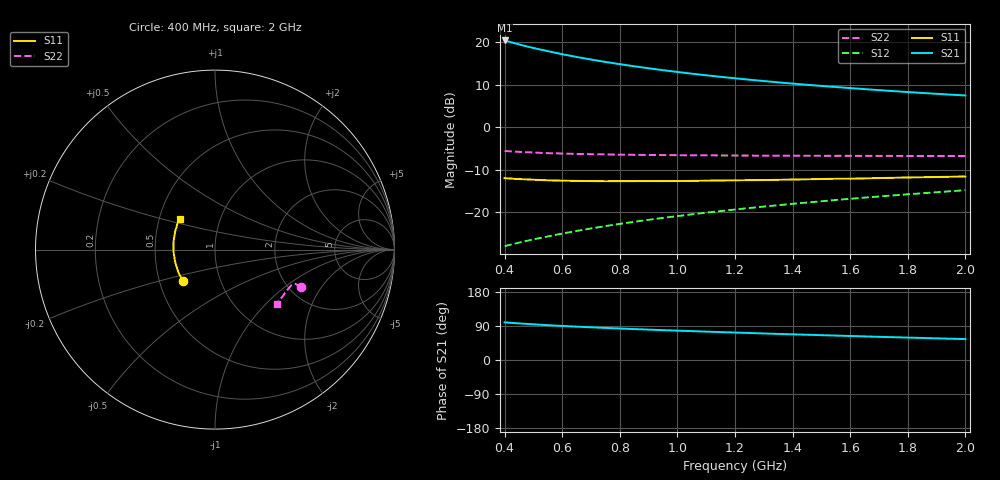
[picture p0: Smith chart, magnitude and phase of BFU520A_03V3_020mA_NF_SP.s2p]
! Filename:  P:\Prog\Test\Noise\ATS_data\Testdata_Net\06 Compressed Noise after Statistics\BFU520A_APG2013_30_A05_03p3V_020mA_NF_CM01_D.sf
! Date/Time: Wed 24/Apr/2013 20:06:17
! BFU520A_APG2013_30_A05_03p3V_1to20mA_NF_CM01_Bias8_R.sf
! Noise Parameter Data File
! BFU520A_APG2013_30_A05_03p3V_1to20mA_NF_CM01
! Date/time: Thu Apr 11 00:04:13 2013
! VAR V_out= 3.301000
! VAR I_out= 19.995000
! VAR V_in= 0.862000
! VAR I_in= 0.236350
! Device data file deembeded for feedlines and parallel
! Original file: \06 Compressed Noise after Statistics\BFU520A_APG2013_30_A05_03p3V_020mA_NF_CM01_R.sf
! Feed-files: PR017V01_150413_Feed1.s2p, PR017V01_150413_Feed2.s2p
! Parallel-file: PR017V01_150413_Par.s2p
# MHz S MA R 50
!  Freq-MHz  S11-mag  S11-arg  S21-mag  S21-arg  S12-mag  S12-arg  S22-mag  S22-arg
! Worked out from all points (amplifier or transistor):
!   37 points, 400 MHz to 2 GHz, reference 50 ohm
!   highest |S21| = 20.4 dB at 400 MHz (marker M1)
!   |S21| within 3 dB of that: start of sweep to 583.6 MHz
!   unconditionally stable (mu >= 1): 665.9 MHz to 1.644 GHz
!   at 500 MHz: K = 0.96, MSG = 22.5 dB, |S12| = -26.5 dB
!   at 1.1 GHz: K = 1.02, MAG = 15.3 dB, |S12| = -20.2 dB
!   at 2 GHz: K = 0.98, MSG = 11.2 dB, |S12| = -14.9 dB
!   lowest NFmin = 1.13 dB at 420 MHz
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400  0.2501 -136.2  10.45 99.4  0.03959 72.2  0.5229 -23.6
420  0.2478 -138.8  10 98.2  0.04118 72.5  0.5172 -23.5
440  0.245 -141.4  9.591 97.1  0.04278 72.8  0.5126 -23.4
460  0.2431 -143.7  9.207 96.1  0.04435 73.1  0.5084 -23.3
480  0.2417 -146.0  8.855 95.1  0.04596 73.3  0.5041 -23.3
500  0.2399 -148.3  8.527 94.2  0.04758 73.5  0.501 -23.2
550  0.2361 -153.5  7.824 91.8  0.05154 74.2  0.4927 -23.1
600  0.2338 -157.9  7.203 89.9  0.05569 74.6  0.4874 -23.2
650  0.2322 -162.0  6.686 88.0  0.05979 74.9  0.4825 -23.4
700  0.2312 -165.8  6.236 86.3  0.06396 75.3  0.4789 -23.6
750  0.2302 -169.3  5.841 84.7  0.06818 75.5  0.4758 -23.9
800  0.2307 -172.5  5.497 83.1  0.07237 75.7  0.4734 -24.3
850  0.2308 -175.8  5.191 81.6  0.07663 75.9  0.4709 -24.7
950  0.2311 178.6  4.67 78.8  0.08516 76.1  0.4676 -25.7
1050  0.2321 173.6  4.249 76.2  0.09376 76.1  0.4648 -26.8
1150  0.2351 168.8  3.901 73.6  0.1025 76.1  0.4627 -28.0
1200  0.2358 166.8  3.749 72.4  0.1069 76.0  0.4622 -28.6
1350  0.2393 160.5  3.358 68.8  0.1203 75.7  0.4606 -30.7
1500  0.2444 154.8  3.047 65.5  0.1338 75.2  0.4585 -32.9
1650  0.2486 149.6  2.795 62.3  0.1476 74.6  0.4579 -35.3
1750  0.2527 146.3  2.649 60.1  0.1568 74.2  0.4571 -36.9
2000  0.2618 138.9  2.352 55.2  0.1804 72.9  0.4561 -41.2
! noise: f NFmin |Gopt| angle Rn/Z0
400  1.168  0.2341  -161.2  0.0979
460  1.139  0.2538  -165.6  0.0897
600  1.274  0.2503  -157.6  0.1018
800  1.235  0.2921  -154.1  0.0891
1000  1.284  0.3133  -146  0.0957
1200  1.341  0.3384  -140.1  0.1033
1400  1.384  0.3562  -133.5  0.1211
1600  1.407  0.3819  -128.9  0.1295
1800  1.44  0.4029  -125.2  0.138
2000  1.514  0.4434  -118.6  0.1525
